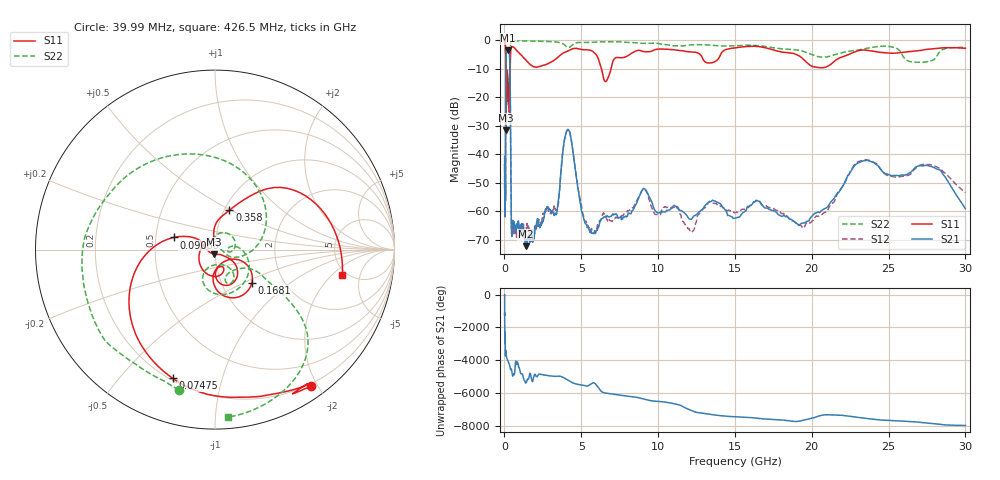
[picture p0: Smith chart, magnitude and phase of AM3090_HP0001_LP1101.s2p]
! Date/Time: Thu, Feb 28, 2019 1:54 PM
! Network Analyzer: Agilent Technologies E8364B Rev: A.07.50.67
! Sweep from 0.010 to 30.000 GHz, 1601 Points, Sweep Type: LOG
! Power Supply: 5.023 V, 0.002 A
# Hz S DB R 50
!freq MagS11 AngS11 MagS21 AngS21 MagS12 AngS12 MagS22 AngS22
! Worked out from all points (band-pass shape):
!   1601 points, 10 MHz to 30 GHz, reference 50 ohm
!   highest |S21| = -3.55 dB at 237.5 MHz (marker M1); lowest = -72.3 dB at 1.382 GHz (marker M2)
!   |S21| within 3 dB of the highest: 101 MHz to 343.8 MHz (242.8 MHz wide, 109 % of centre)
!   lowest |S11| = -31.6 dB at 98.93 MHz (marker M3), VSWR 1.05, Z = 49.5 - j2.57 ohm
!   |S11| at or under -10 dB: 89.62 MHz to 369.6 MHz (280 MHz wide, 122 % of centre); 6.309 GHz to 6.936 GHz (626.8 MHz wide, 9.46 % of centre)
!   |S22| runs from -33.5 to -0.1 dB; largest |S21 - S12| = 0.015
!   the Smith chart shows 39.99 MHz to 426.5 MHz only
!   S11 on the Smith chart (normalised r, x): 39.99 MHz: 0.17, -1.91; 74.75 MHz: 0.21, -0.70; 90.86 MHz: 0.62, +0.09; 168.1 MHz: 1.39, -0.55; 358 MHz: 1.06, +0.49; 426.5 MHz: 4.59, -2.70
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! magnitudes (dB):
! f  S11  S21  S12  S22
! 10 MHz  -0.2  -40.8  -45.0  -0.6
! 38.04 MHz  -0.5  -61.1  -60.2  -1.7
! 39.99 MHz  -0.6  -60.8  -59.8  -1.9
! 74.75 MHz  -2.4  -47.9  -45.7  -4.3
! 90.86 MHz  -12.4  -14.1  -14.1  -12.9
! 98.93 MHz  -31.6  -7.2  -7.2  -33.2
! 114.4 MHz  -13.7  -4.8  -4.8  -19.2
! 144.7 MHz  -19.5  -3.6  -3.6  -22.2
! 168.1 MHz  -11.2  -3.6  -3.6  -13.7
! 237.5 MHz  -19.9  -3.6  -3.5  -18.4
! 358 MHz  -12.6  -8.7  -8.7  -8.5
! 426.5 MHz  -2.8  -54.0  -53.5  -0.6
! 550.5 MHz  -2.4  -64.7  -66.3  -0.2
! 1.382 GHz  -6.8  -72.3  -68.3  -0.3
! 2.084 GHz  -9.5  -64.3  -65.7  -0.4
! 3.352 GHz  -6.6  -61.3  -59.7  -0.7
! 4.115 GHz  -3.9  -31.4  -31.4  -2.5
! 5.446 GHz  -3.4  -65.6  -65.2  -0.8
! 7.926 GHz  -5.8  -62.1  -60.5  -0.8
! 19.41 GHz  -6.5  -64.2  -66.0  -3.9
! 23.48 GHz  -3.5  -42.3  -42.0  -3.0
! 30 GHz  -2.8  -59.2  -53.5  -2.5
